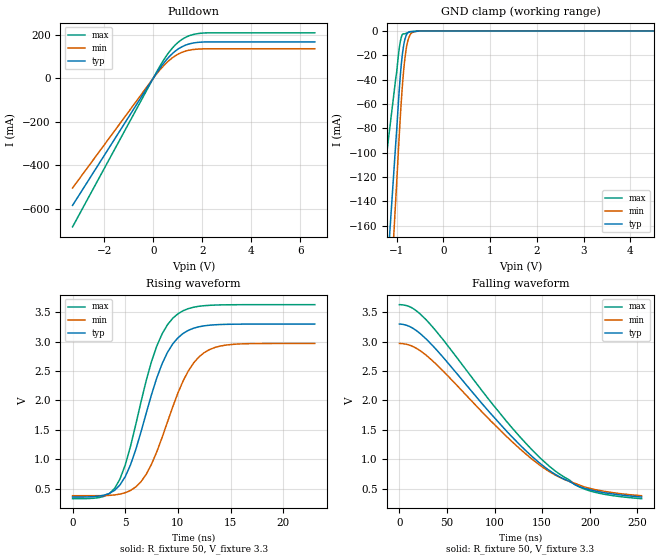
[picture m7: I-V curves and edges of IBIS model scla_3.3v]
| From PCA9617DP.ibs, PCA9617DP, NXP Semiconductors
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[Model]   scla_3.3v
Model_type Open_drain
Vref=3.300E+00
Rref=1.350E+03
Cref=5.000E-11
Vmeas=1.650E+00
C_comp   9.000E-13   8.790E-13   9.210E-13
[Voltage Range]   3.300E+00   2.970E+00   3.630E+00
[POWER Clamp Reference]   3.300E+00   2.970E+00   3.630E+00
[GND Clamp Reference]   0.000E+00   0.000E+00   0.000E+00
[Pullup Reference]   3.300E+00   2.970E+00   3.630E+00
[Pulldown Reference]   0.000E+00   0.000E+00   0.000E+00
[Temperature Range]   25   85   -40
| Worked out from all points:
|   slope of the pulldown table from 0 to 0.495 V, typ, clamps not added: 6.28 ohm
|   GND clamp passes 1 mA (typ) near -0.74 V on its own axis
|   rising waveform, R_fixture 50, V_fixture 3.3: 20-80 % time 3.15ns typ, 3.4ns min, 2.96ns max; typ from 0.357 V to 3.3 V
|   falling waveform, R_fixture 50, V_fixture 3.3: 20-80 % time 99.4ns typ, 98.7ns min, 101ns max; typ from 3.3 V to 0.357 V
[GND Clamp]
-3.3V     -1.407A    -1.729A    -767.3mA
-1.02V    -92.4mA    -138.6mA   -39.06mA
-1V       -81.63mA   -125mA     -33.78mA
-940mV    -45.74mA   -82.48mA   -12.86mA
-900mV    -26.95mA   -57.17mA   -5.047mA
-860mV    -13.99mA   -36.47mA   -2.379mA
-820mV    -6.297mA   -21.19mA   -2.219mA
-800mV    -3.963mA   -15.56mA   -1.933mA
-760mV    -1.317mA   -7.791mA   -1.258mA
-700mV    -521.9uA   -2.253mA   -534.1uA
-540mV    -141.3uA   -82.32uA   -28.38uA
6.6V      0A         0A         0A
[Pulldown]
-3.3V     -584.7mA   -504.8mA   -683.5mA
180mV     31.04mA    25.97mA    37.45mA
620mV     95.08mA    78.98mA    116.1mA
820mV     117mA      96.83mA    143.3mA
1.06V     137.2mA    113.2mA    168.8mA
1.48V     157.8mA    129mA      195.5mA
2.04V     166.1mA    134.8mA    207.4mA
6.6V      166.7mA    135.2mA    208.4mA
[Rising Waveform]
R_fixture = 50
V_fixture = 3.3
V_fixture_min = 2.97
V_fixture_max = 3.63
0s        357.5mV    379.7mV    329.3mV
3ns       389.4mV    381.7mV    369.7mV
4.5ns     562.8mV    407.3mV    662.9mV
5.5ns     904.4mV    469mV      1.218V
6.5ns     1.466V     618.2mV    1.976V
8ns       2.385V     1.127V     2.927V
10ns      3.065V     2.124V     3.474V
11.5ns    3.23V      2.639V     3.587V
13.5ns    3.287V     2.901V     3.623V
23ns      3.3V       2.97V      3.63V
[Falling Waveform]
R_fixture = 50
V_fixture = 3.3
V_fixture_min = 2.97
V_fixture_max = 3.63
0s        3.3V       2.97V      3.63V
14ns      3.23V      2.92V      3.568V
29.5ns    3.023V     2.751V     3.348V
114ns     1.454V     1.366V     1.617V
139.5ns   1.045V     999.2mV    1.158V
161ns     771.1mV    755.6mV    834.8mV
185.5ns   559.7mV    584mV      559.2mV
197.5ns   492.2mV    515mV      475.1mV
221.5ns   415.4mV    438.5mV    387.7mV
254.5ns   357.5mV    379.7mV    329.3mV
[Ramp]
dV/dt_r   1.7655E+00/3.1280E-09   1.5542E+00/3.3830E-09   1.9804E+00/2.9420E-09
dV/dt_f   1.7655E+00/9.9405E-08   1.5542E+00/9.8719E-08   1.9804E+00/1.0104E-07
R_load = 50
